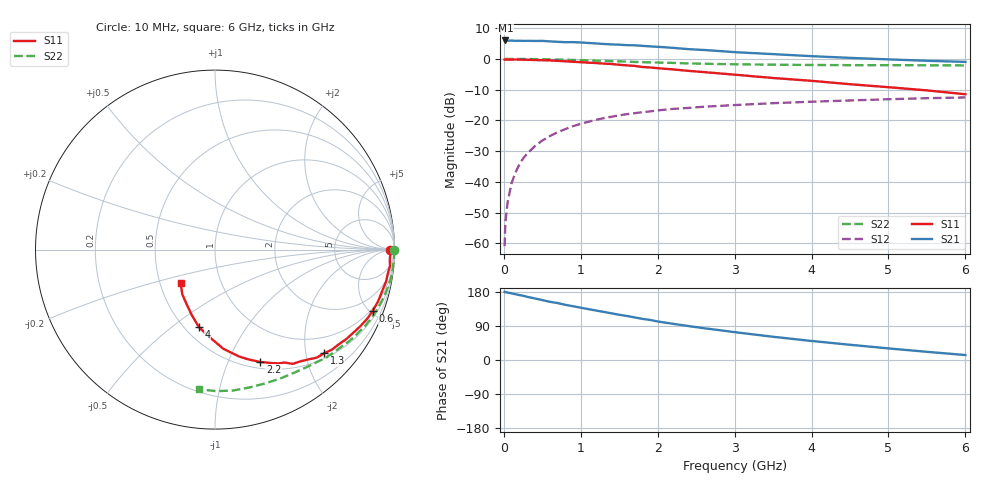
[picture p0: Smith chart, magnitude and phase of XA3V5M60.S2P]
! SIEMENS Discrete & RF Semiconductors
! BFY180
! Si NPN RF Bipolar Junction Transistor in MICRO-X
! VCE = 3.5 V  IC = 0.6 mA
! Common Emitter S-Parameters:  May  1997
# GHz  S  MA  R  50
!  f  S11  S21  S12  S22
! GHz  MAG  ANG  MAG  ANG  MAG  ANG  MAG  ANG
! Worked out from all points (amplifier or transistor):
!   36 points, 10 MHz to 6 GHz, reference 50 ohm
!   highest |S21| = 6.0 dB at 20 MHz (marker M1)
!   |S21| within 3 dB of that: start of sweep to 2.528 GHz
!   unconditionally stable (mu >= 1): 5.171 GHz to end of sweep
!   at 250 MHz: K = 0.04, MSG = 19.1 dB, |S12| = -32.4 dB
!   at 1.4 GHz: K = 0.41, MSG = 11.8 dB, |S12| = -18.8 dB
!   at 6 GHz: K = 1.03, MAG = 4.6 dB, |S12| = -12.5 dB
!   S11 on the Smith chart (normalised r, x): 10 MHz: 81, -12; 600 MHz: 0.84, -5.19; 1.3 GHz: 0.61, -2.37; 2.2 GHz: 0.57, -1.32; 4 GHz: 0.59, -0.63; 6 GHz: 0.64, -0.26
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0.01  0.9762 -0.2  1.986 179.8  0.0009 93.6  0.9988 -0.2
0.02  0.9724 -0.6  1.997 179.0  0.0022 98.2  0.9999 -0.4
0.05  0.9765 -1.7  1.97 178.0  0.0047 87.8  0.9993 -1.1
0.1  0.9757 -3.5  1.989 175.9  0.0095 87.8  0.998 -2.4
0.2  0.9739 -7.0  1.976 171.4  0.019 84.6  0.996 -4.7
0.25  0.9707 -9.0  1.967 169.5  0.024 84.6  0.9972 -6.0
0.4  0.9592 -14.1  1.962 162.6  0.0379 79.3  0.9929 -9.3
0.5  0.9533 -17.6  1.965 158.1  0.047 76.6  0.9869 -11.7
0.6  0.943 -21.3  1.927 153.5  0.0557 74.2  0.9816 -14.0
0.9  0.8982 -31.2  1.875 141.9  0.0806 66.1  0.9619 -20.6
1.1  0.8683 -37.4  1.817 134.2  0.095 61.6  0.9467 -24.8
1.3  0.8381 -43.6  1.751 126.9  0.1089 56.9  0.9281 -28.9
1.7  0.7697 -55.8  1.666 112.4  0.1309 49.0  0.8929 -36.3
2  0.7069 -63.4  1.575 101.7  0.1455 43.9  0.8734 -41.4
2.2  0.6754 -68.0  1.514 95.5  0.1539 40.5  0.8615 -44.7
2.6  0.6108 -77.2  1.398 83.9  0.1668 35.1  0.8356 -50.6
2.8  0.5822 -81.0  1.344 78.8  0.1723 32.6  0.8259 -53.4
3.5  0.4895 -93.4  1.197 61.3  0.1907 25.0  0.8054 -62.7
4  0.4404 -101.8  1.109 50.2  0.2015 20.0  0.7967 -69.2
4.5  0.3878 -109.4  1.04 40.2  0.211 15.8  0.7918 -75.9
5.5  0.3079 -126.4  0.933 21.6  0.2298 7.0  0.7886 -89.7
6  0.2664 -135.9  0.895 13.1  0.2365 2.5  0.7824 -96.7
